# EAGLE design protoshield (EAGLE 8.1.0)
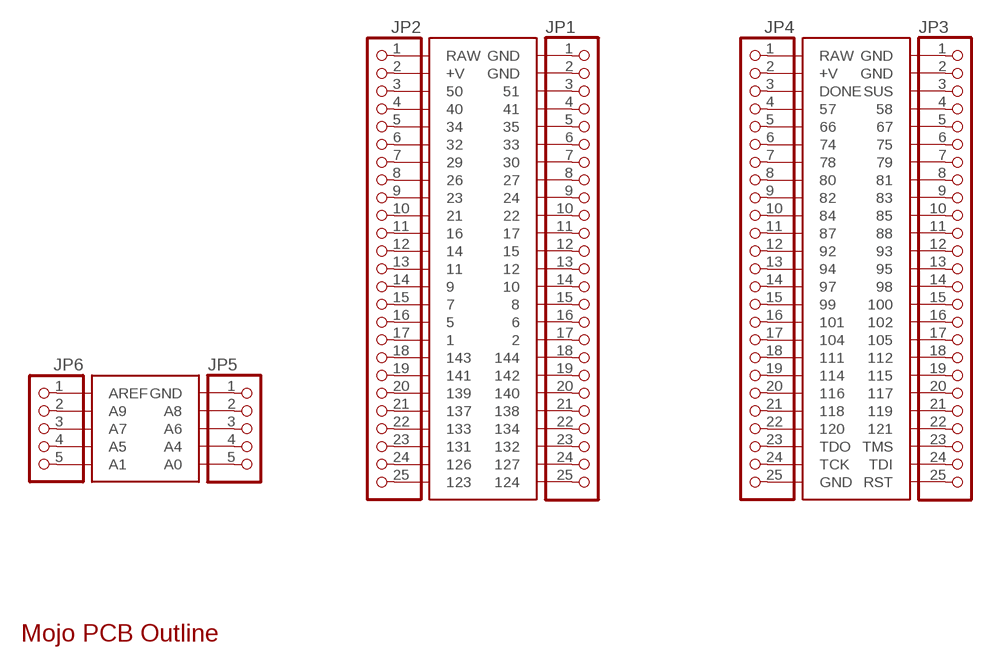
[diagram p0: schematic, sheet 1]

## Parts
JP1  PINHD-1X25  [1X25]
JP2  PINHD-1X25  [1X25]
JP3  PINHD-1X25  [1X25]
JP4  PINHD-1X25  [1X25]
JP5  PINHD-1X5MOJO  [1X5]
JP6  PINHD-1X5MOJO  [1X5]
U$1  MOJO_V2V3_NO_LABEL  [MOJO_V3_NO_LABEL]
U$2  MOJO_OUTLINE  [MOJO_OUTLINE]

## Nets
N$1: JP5.1 U$1.GND@5(GND)
N$2: JP5.2 U$1.A8
N$3: JP5.3 U$1.A6
N$4: JP5.4 U$1.A4
N$5: JP5.5 U$1.A0
N$6: JP6.1 U$1.AREF
N$7: JP6.2 U$1.A9
N$8: JP6.3 U$1.A7
N$9: JP6.4 U$1.A5
N$10: JP6.5 U$1.A1
N$11: JP1.1 U$1.GND@1(GND)
N$12: JP1.2 U$1.GND@2(GND)
N$13: JP1.3 U$1.51
N$14: JP1.4 U$1.41
N$15: JP1.5 U$1.35
N$16: JP1.6 U$1.33
N$17: JP1.7 U$1.30
N$18: JP1.8 U$1.27
N$19: JP1.9 U$1.24
N$20: JP1.10 U$1.22
N$21: JP1.11 U$1.17
N$22: JP1.12 U$1.15
N$23: JP1.13 U$1.12
N$24: JP1.14 U$1.10
N$25: JP1.15 U$1.8
N$26: JP1.16 U$1.6
N$27: JP1.17 U$1.2
N$28: JP1.18 U$1.144
N$29: JP1.19 U$1.142
N$30: JP1.20 U$1.140
N$31: JP1.21 U$1.138
N$32: JP1.22 U$1.134
N$33: JP1.23 U$1.132
N$34: JP1.24 U$1.127
N$35: JP1.25 U$1.124
N$36: JP2.1 U$1.RAW@1(RAW)
N$37: JP2.2 U$1.V@1(+V)
N$38: JP2.3 U$1.50
N$39: JP2.4 U$1.40
N$40: JP2.5 U$1.34
N$41: JP2.6 U$1.32
N$42: JP2.7 U$1.29
N$43: JP2.8 U$1.26
N$44: JP2.9 U$1.23
N$45: JP2.10 U$1.21
N$46: JP2.11 U$1.16
N$47: JP2.12 U$1.14
N$48: JP2.13 U$1.11
N$49: JP2.14 U$1.9
N$50: JP2.15 U$1.7
N$51: JP2.16 U$1.5
N$52: JP2.17 U$1.1
N$53: JP2.18 U$1.143
N$54: JP2.19 U$1.141
N$55: JP2.20 U$1.139
N$56: JP2.21 U$1.137
N$57: JP2.22 U$1.133
N$58: JP2.23 U$1.131
N$59: JP2.24 U$1.126
N$60: JP2.25 U$1.123
N$61: JP3.1 U$1.GND@3(GND)
N$62: JP3.2 U$1.GND@4(GND)
N$63: JP3.3 U$1.SUS
N$64: JP3.4 U$1.58
N$65: JP3.5 U$1.67
N$66: JP3.6 U$1.75
N$67: JP3.7 U$1.79
N$68: JP3.8 U$1.81
N$69: JP3.9 U$1.83
N$70: JP3.10 U$1.85
N$71: JP3.11 U$1.88
N$72: JP3.12 U$1.93
N$73: JP3.13 U$1.95
N$74: JP3.14 U$1.98
N$75: JP3.15 U$1.100
N$76: JP3.16 U$1.102
N$77: JP3.17 U$1.105
N$78: JP3.18 U$1.112
N$79: JP3.19 U$1.115
N$80: JP3.20 U$1.117
N$81: JP3.21 U$1.119
N$82: JP3.22 U$1.121
N$83: JP3.23 U$1.TMS
N$84: JP3.24 U$1.TDI
N$85: JP3.25 U$1.RST
N$86: JP4.1 U$1.RAW@2(RAW)
N$87: JP4.2 U$1.V@2(+V)
N$88: JP4.3 U$1.DONE
N$89: JP4.4 U$1.57
N$90: JP4.5 U$1.66
N$91: JP4.6 U$1.74
N$92: JP4.7 U$1.78
N$93: JP4.8 U$1.80
N$94: JP4.9 U$1.82
N$95: JP4.10 U$1.84
N$96: JP4.11 U$1.87
N$97: JP4.12 U$1.92
N$98: JP4.13 U$1.94
N$99: JP4.14 U$1.97
N$100: JP4.15 U$1.99
N$101: JP4.16 U$1.101
N$102: JP4.17 U$1.104
N$103: JP4.18 U$1.111
N$104: JP4.19 U$1.114
N$105: JP4.20 U$1.116
N$106: JP4.21 U$1.118
N$107: JP4.22 U$1.120
N$108: JP4.23 U$1.TDO
N$109: JP4.24 U$1.TCK
N$110: JP4.25 U$1.GND@6(GND)

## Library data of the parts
JP1-JP4 = embeddedmicro:PINHD-1X25: PIN HEADER
JP5 JP6 = embeddedmicro:PINHD-1X5: PIN HEADER
U$1 = embeddedmicro:MOJO_V2
U$2 = embeddedmicro:MOJO_OUTLINE

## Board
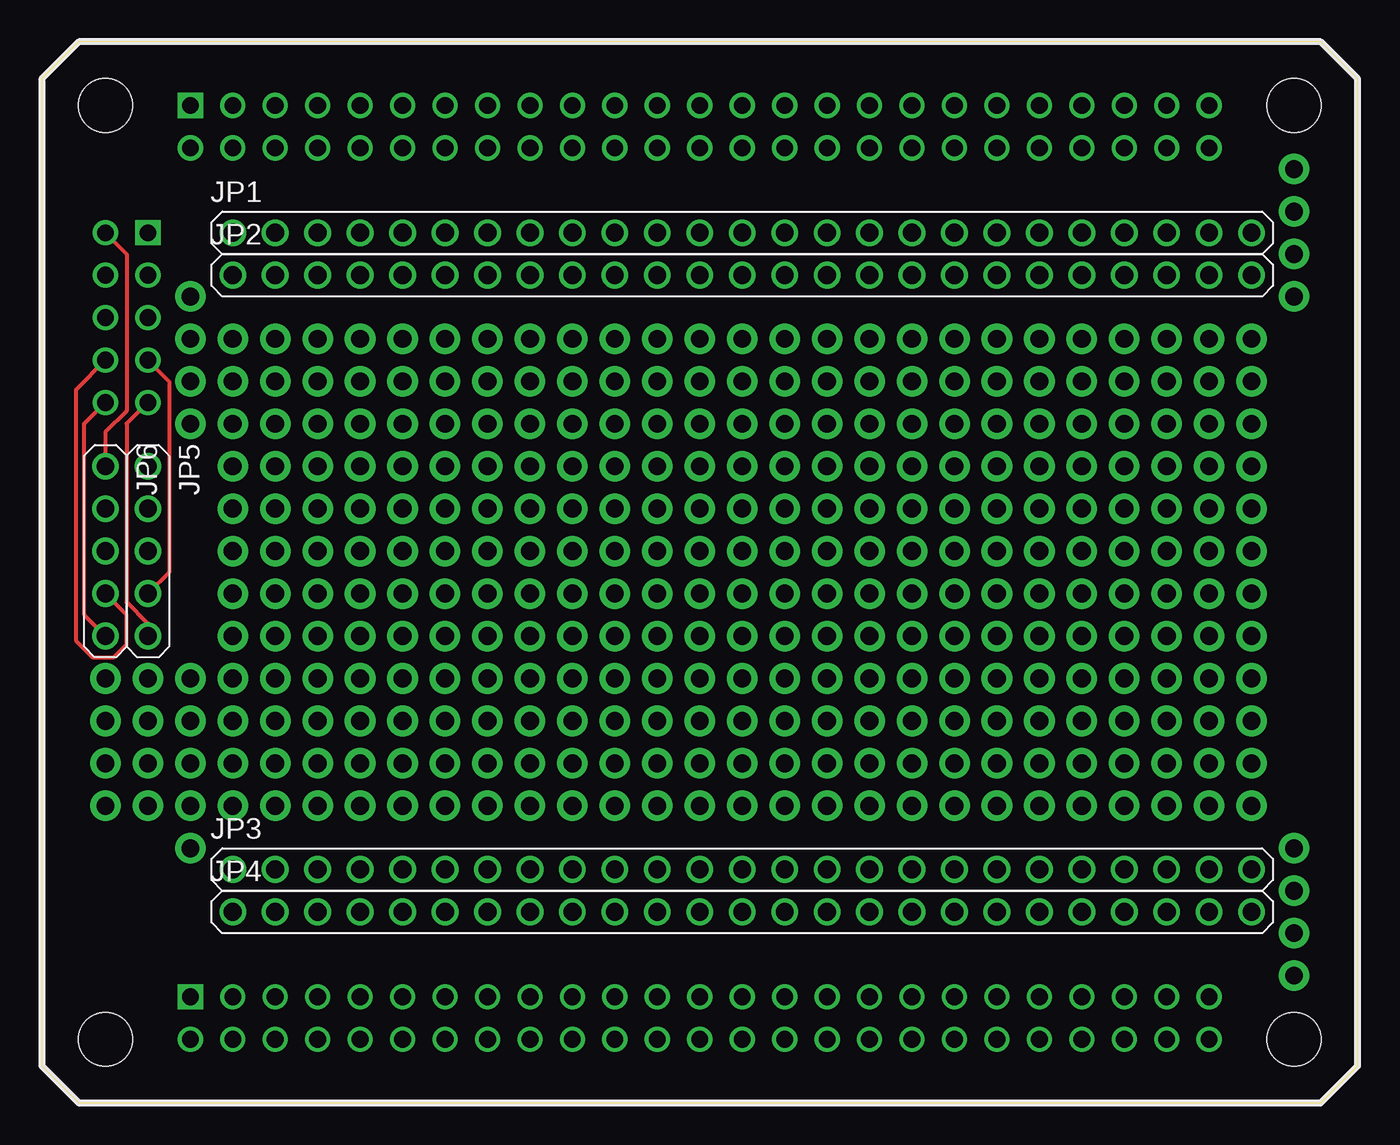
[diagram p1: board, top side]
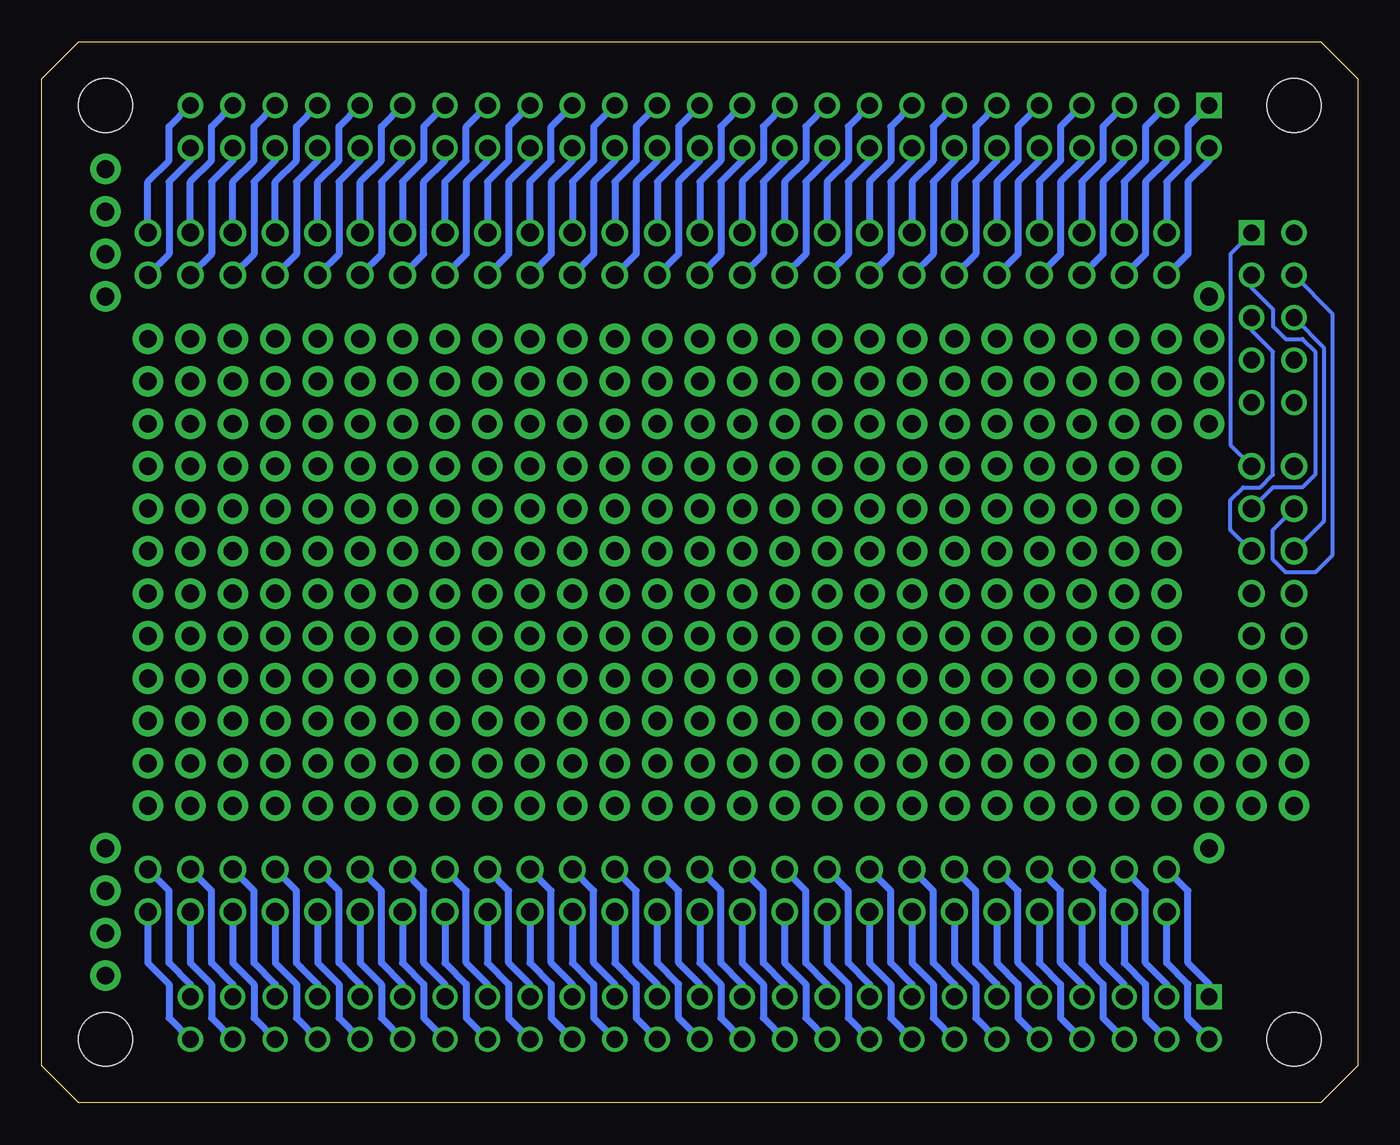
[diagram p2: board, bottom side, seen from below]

Size 78.74 x 63.5 mm. Coordinates in mm from the lower left corner, seen from the top.
Copper layers (1*16): Top 0.035mm / dielectric 1.5mm / Bottom 0.035mm
Design rules "default *": minimum track width 10mil, minimum drill 24mil, track to track 8mil, track to pad 8mil, pad to pad 8mil, via to via 8mil, smd to smd 8mil, copper to edge 40mil, drill to drill 8mil, minimum pad ring 10mil, minimum via ring 15mil, stop-mask expansion 4mil, vias tented up to drill 0mil, thermal gap 10mil

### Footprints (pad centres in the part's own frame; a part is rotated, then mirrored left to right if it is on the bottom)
1X25 = drill 1.067: 1 -29.21,0; 2 -26.67,0; 3 -24.13,0; 4 -21.59,0; 5 -19.05,0; 6 -16.51,0; 7 -13.97,0; 8 -11.43,0; 9 -8.89,0; 10 -6.35,0; 11 -3.81,0; 12 -1.27,0; 13 1.27,0; 14 3.81,0; 15 6.35,0; 16 8.89,0; 17 11.43,0; 18 13.97,0; 19 16.51,0; 20 19.05,0; 21 21.59,0; 22 24.13,0; 23 26.67,0; 24 29.21,0; 25 31.75,0
1X5 = drill 1.067: 1 -5.08,0; 2 -2.54,0; 3 0,0; 4 2.54,0; 5 5.08,0
MOJO_V3_NO_LABEL = drill 1: 1 49.53,57.15; 2 49.53,59.69; 5 46.99,57.15; 6 46.99,59.69; 7 44.45,57.15; 8 44.45,59.69; 9 41.91,57.15; 10 41.91,59.69; 11 39.37,57.15; 12 39.37,59.69; 14 36.83,57.15; 15 36.83,59.69; 16 34.29,57.15; 17 34.29,59.69; 21 31.75,57.15; 22 31.75,59.69; 23 29.21,57.15; 24 29.21,59.69; 26 26.67,57.15; 27 26.67,59.69; 29 24.13,57.15; 30 24.13,59.69; 32 21.59,57.15; 33 21.59,59.69; 34 19.05,57.15; 35 19.05,59.69; 40 16.51,57.15; 41 16.51,59.69; 50 13.97,57.15; 51 13.97,59.69; 57 16.51,3.81; 58 16.51,6.35; 66 19.05,3.81; 67 19.05,6.35; 74 21.59,3.81; 75 21.59,6.35; 78 24.13,3.81; 79 24.13,6.35; 80 26.67,3.81; 81 26.67,6.35; 82 29.21,3.81; 83 29.21,6.35; 84 31.75,3.81; 85 31.75,6.35; 87 34.29,3.81; 88 34.29,6.35; 92 36.83,3.81; 93 36.83,6.35; 94 39.37,3.81; 95 39.37,6.35; 97 41.91,3.81; 98 41.91,6.35; 99 44.45,3.81; 100 44.45,6.35; 101 46.99,3.81; 102 46.99,6.35; 104 49.53,3.81; 105 49.53,6.35; 111 52.07,3.81; 112 52.07,6.35; 114 54.61,3.81; 115 54.61,6.35; 116 57.15,3.81; 117 57.15,6.35; 118 59.69,3.81; 119 59.69,6.35; 120 62.23,3.81; 121 62.23,6.35; 123 69.85,57.15; 124 69.85,59.69; 126 67.31,57.15; 127 67.31,59.69; 131 64.77,57.15; 132 64.77,59.69; 133 62.23,57.15; 134 62.23,59.69; 137 59.69,57.15; 138 59.69,59.69; 139 57.15,57.15; 140 57.15,59.69; 141 54.61,57.15; 142 54.61,59.69; 143 52.07,57.15; 144 52.07,59.69; A0 6.35,41.91; A1 3.81,41.91; A4 6.35,44.45; A5 3.81,44.45; A6 6.35,46.99; A7 3.81,46.99; A8 6.35,49.53; A9 3.81,49.53; AREF 3.81,52.07; DONE 13.97,3.81; GND@2 11.43,59.69; GND@4 11.43,6.35; GND@6 69.85,3.81; RAW@1 8.89,57.15; RAW@2 8.89,3.81; RST 69.85,6.35; SUS 13.97,6.35; TCK 67.31,3.81; TDI 67.31,6.35; TDO 64.77,3.81; TMS 64.77,6.35; V@1 11.43,57.15; V@2 11.43,3.81 | drill 1 square: GND@1 8.89,59.69; GND@3 8.89,6.35; GND@5 6.35,52.07 | hole 3.2: 3.81,3.81; 3.81,59.69; 74.93,59.69; 74.93,3.81

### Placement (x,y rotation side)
JP1  40.64,52.07 0 top
JP2  40.64,49.53 0 top
JP3  40.64,13.97 0 top
JP4  40.64,11.43 0 top
JP5  6.35,33.02 270 top
JP6  3.81,33.02 270 top
U$1  0,0 0 top
U$2  0,0 0 top

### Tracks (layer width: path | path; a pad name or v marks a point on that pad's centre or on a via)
N$1
  Bottom 0.254: U$1.GND@5 7.62,50.8 7.62,39.37 JP5.1
N$2
  Bottom 0.254: U$1.A8 6.35,48.77 5.08,47.5 5.08,46.48 4.32,45.72 3.3,45.72 2.54,44.96 2.54,37.59 3.3,36.83 5.08,36.83 JP5.2
N$3
  Bottom 0.254: JP5.3 7.62,34.29 7.62,36.07 6.86,36.83 5.84,36.83 5.08,37.59 5.08,44.96 6.35,46.23 U$1.A6
N$4
  Top 0.254: U$1.A4 7.62,43.18 7.62,31.75 JP5.4
N$5
  Top 0.254: U$1.A0 5.08,40.64 5.08,29.97 6.35,28.7 JP5.5
N$6
  Top 0.254: U$1.AREF 4.83,51.05 5.08,50.8 5.08,41.4 3.81,40.13 JP6.1
N$7
  Bottom 0.254: U$1.A9 1.52,47.24 1.52,32.77 2.54,31.75 4.32,31.75 5.08,32.51 5.08,34.29 JP6.2
N$8
  Bottom 0.254: U$1.A7 2.03,45.21 2.03,34.8 JP6.3
N$9
  Top 0.254: U$1.A5 2.03,42.67 2.03,27.69 3.05,26.67 4.32,26.67 5.08,27.43 5.08,29.21 JP6.4
N$10
  Top 0.254: U$1.A1 2.54,40.64 2.54,29.21 JP6.5
N$11
  Bottom 0.406: U$1.GND@1 10.16,58.42 10.16,56.39 11.43,55.12 JP1.1
N$12
  Bottom 0.406: U$1.GND@2 12.7,58.42 12.7,56.39 13.97,55.12 JP1.2
N$13
  Bottom 0.406: U$1.51 15.24,58.42 15.24,56.39 16.51,55.12 JP1.3
N$14
  Bottom 0.406: U$1.41 17.78,58.42 17.78,56.39 19.05,55.12 JP1.4
N$15
  Bottom 0.406: U$1.35 20.32,58.42 20.32,56.39 21.59,55.12 JP1.5
N$16
  Bottom 0.406: U$1.33 22.86,58.42 22.86,56.39 24.13,55.12 JP1.6
N$17
  Bottom 0.406: U$1.30 25.4,58.42 25.4,56.39 26.67,55.12 JP1.7
N$18
  Bottom 0.406: U$1.27 27.94,58.42 27.94,56.39 29.21,55.12 JP1.8
N$19
  Bottom 0.406: U$1.24 30.48,58.42 30.48,56.39 31.75,55.12 JP1.9
N$20
  Bottom 0.406: U$1.22 33.02,58.42 33.02,56.39 34.29,55.12 JP1.10
N$21
  Bottom 0.406: U$1.17 35.56,58.42 35.56,56.39 36.83,55.12 JP1.11
N$22
  Bottom 0.406: U$1.15 38.1,58.42 38.1,56.39 39.37,55.12 JP1.12
N$23
  Bottom 0.406: U$1.12 40.64,58.42 40.64,56.39 41.91,55.12 JP1.13
N$24
  Bottom 0.406: U$1.10 43.18,58.42 43.18,56.39 44.45,55.12 JP1.14
N$25
  Bottom 0.406: U$1.8 45.72,58.42 45.72,56.39 46.99,55.12 JP1.15
N$26
  Bottom 0.406: JP1.16 49.53,55.12 48.26,56.39 48.26,58.42 U$1.6
N$27
  Bottom 0.406: U$1.2 50.8,58.42 50.8,56.39 52.07,55.12 JP1.17
N$28
  Bottom 0.406: JP1.18 54.61,55.12 53.34,56.39 53.34,58.42 U$1.144
N$29
  Bottom 0.406: U$1.142 55.88,58.42 55.88,56.39 57.15,55.12 JP1.19
N$30
  Bottom 0.406: JP1.20 59.69,55.12 58.42,56.39 58.42,58.42 U$1.140
N$31
  Bottom 0.406: JP1.21 62.23,55.12 60.96,56.39 60.96,58.42 U$1.138
N$32
  Bottom 0.406: JP1.22 64.77,55.12 63.5,56.39 63.5,58.42 U$1.134
N$33
  Bottom 0.406: JP1.23 67.31,55.12 66.04,56.39 66.04,58.42 U$1.132
N$34
  Bottom 0.406: JP1.24 69.85,55.12 68.58,56.39 68.58,58.42 U$1.127
N$35
  Bottom 0.406: JP1.25 72.39,55.12 71.12,56.39 71.12,58.42 U$1.124
N$36
  Bottom 0.406: U$1.RAW@1 8.89,56.39 10.16,55.12 10.16,50.8 JP2.1
N$37
  Bottom 0.406: U$1.V@1 11.43,56.39 12.7,55.12 12.7,50.8 JP2.2
N$38
  Bottom 0.406: U$1.50 13.97,56.39 15.24,55.12 15.24,50.8 JP2.3
N$39
  Bottom 0.406: U$1.40 16.51,56.39 17.78,55.12 17.78,50.8 JP2.4
N$40
  Bottom 0.406: U$1.34 19.05,56.39 20.32,55.12 20.32,50.8 JP2.5
N$41
  Bottom 0.406: U$1.32 21.59,56.39 22.86,55.12 22.86,50.8 JP2.6
N$42
  Bottom 0.406: U$1.29 24.13,56.39 25.4,55.12 25.4,50.8 JP2.7
N$43
  Bottom 0.406: U$1.26 26.67,56.39 27.94,55.12 27.94,50.8 JP2.8
N$44
  Bottom 0.406: U$1.23 29.21,56.39 30.23,55.37 30.48,55.12 30.48,50.8 JP2.9
N$45
  Bottom 0.406: U$1.21 31.75,56.39 33.02,55.12 33.02,50.8 JP2.10
N$46
  Bottom 0.406: U$1.16 34.29,56.39 35.31,55.37 35.56,55.12 35.56,50.8 JP2.11
N$47
  Bottom 0.406: U$1.14 36.83,56.39 38.1,55.12 38.1,50.8 JP2.12
N$48
  Bottom 0.406: U$1.11 39.37,56.39 40.64,55.12 40.64,50.8 JP2.13
N$49
  Bottom 0.406: U$1.9 41.91,56.39 43.18,55.12 43.18,50.8 JP2.14
N$50
  Bottom 0.406: U$1.7 44.45,56.39 45.72,55.12 45.72,50.8 JP2.15
N$51
  Bottom 0.406: U$1.5 46.99,56.39 48.26,55.12 48.26,50.8 JP2.16
N$52
  Bottom 0.406: U$1.1 49.53,56.39 50.8,55.12 50.8,50.8 JP2.17
N$53
  Bottom 0.406: U$1.143 52.07,56.39 53.34,55.12 53.34,50.8 JP2.18
N$54
  Bottom 0.406: JP2.19 55.88,50.8 55.88,55.12 54.61,56.39 U$1.141
N$55
  Bottom 0.406: U$1.139 57.15,56.39 58.17,55.37 58.42,55.12 58.42,50.8 JP2.20
N$56
  Bottom 0.406: U$1.137 59.69,56.39 60.96,55.12 60.96,50.8 JP2.21
N$57
  Bottom 0.406: U$1.133 62.23,56.39 63.5,55.12 63.5,50.8 JP2.22
N$58
  Bottom 0.406: U$1.131 64.77,56.39 66.04,55.12 66.04,50.8 JP2.23
N$59
  Bottom 0.406: U$1.126 67.31,56.39 68.58,55.12 68.58,50.8 JP2.24
N$60
  Bottom 0.406: U$1.123 69.85,56.39 71.12,55.12 71.12,50.8 JP2.25
N$61
  Bottom 0.406: U$1.GND@3 8.89,7.11 10.16,8.38 10.16,12.7 JP3.1
N$62
  Bottom 0.406: U$1.GND@4 11.43,7.11 12.7,8.38 12.7,12.7 JP3.2
N$63
  Bottom 0.406: U$1.SUS 13.97,7.11 15.24,8.38 15.24,12.7 JP3.3
N$64
  Bottom 0.406: U$1.58 16.51,7.11 17.78,8.38 17.78,12.7 JP3.4
N$65
  Bottom 0.406: U$1.67 19.05,7.11 20.32,8.38 20.32,12.7 JP3.5
N$66
  Bottom 0.406: U$1.75 21.59,7.11 22.86,8.38 22.86,12.7 JP3.6
N$67
  Bottom 0.406: U$1.79 24.13,7.11 25.4,8.38 25.4,12.7 JP3.7
N$68
  Bottom 0.406: U$1.81 26.67,7.11 27.94,8.38 27.94,12.7 JP3.8
N$69
  Bottom 0.406: U$1.83 29.21,7.11 30.48,8.38 30.48,12.7 JP3.9
N$70
  Bottom 0.406: U$1.85 31.75,7.11 33.02,8.38 33.02,12.7 JP3.10
N$71
  Bottom 0.406: U$1.88 34.29,7.11 35.56,8.38 35.56,12.7 JP3.11
N$72
  Bottom 0.406: U$1.93 36.83,7.11 38.1,8.38 38.1,12.7 JP3.12
N$73
  Bottom 0.406: U$1.95 39.37,7.11 40.39,8.13 40.64,8.38 40.64,12.7 JP3.13
N$74
  Bottom 0.406: U$1.98 41.91,7.11 43.18,8.38 43.18,12.7 JP3.14
N$75
  Bottom 0.406: U$1.100 44.45,7.11 45.72,8.38 45.72,12.7 JP3.15
N$76
  Bottom 0.406: U$1.102 46.99,7.11 48.26,8.38 48.26,12.7 JP3.16
N$77
  Bottom 0.406: U$1.105 49.53,7.11 50.8,8.38 50.8,12.7 JP3.17
N$78
  Bottom 0.406: U$1.112 52.07,7.11 53.34,8.38 53.34,12.7 JP3.18
N$79
  Bottom 0.406: U$1.115 54.61,7.11 55.88,8.38 55.88,12.7 JP3.19
N$80
  Bottom 0.406: U$1.117 57.15,7.11 58.42,8.38 58.42,12.7 JP3.20
N$81
  Bottom 0.406: U$1.119 59.69,7.11 60.96,8.38 60.96,12.7 JP3.21
N$82
  Bottom 0.406: U$1.121 62.23,7.11 63.25,8.13 63.5,8.38 63.5,12.7 JP3.22
N$83
  Bottom 0.406: U$1.TMS 64.77,7.11 66.04,8.38 66.04,12.7 JP3.23
N$84
  Bottom 0.406: U$1.TDI 67.31,7.11 68.58,8.38 68.58,12.7 JP3.24
N$85
  Bottom 0.406: U$1.RST 69.85,7.11 71.12,8.38 71.12,12.7 JP3.25
N$86
  Bottom 0.406: U$1.RAW@2 10.16,5.08 10.16,7.11 11.43,8.38 JP4.1
N$87
  Bottom 0.406: JP4.2 13.97,8.38 12.7,7.11 12.7,5.08 U$1.V@2
N$88
  Bottom 0.406: JP4.3 16.51,8.38 15.24,7.11 15.24,5.08 U$1.DONE
N$89
  Bottom 0.406: JP4.4 19.05,8.38 17.78,7.11 17.78,5.08 U$1.57
N$90
  Bottom 0.406: JP4.5 21.59,8.38 20.32,7.11 20.32,5.08 U$1.66
N$91
  Bottom 0.406: JP4.6 24.13,8.38 22.86,7.11 22.86,5.08 U$1.74
N$92
  Bottom 0.406: JP4.7 26.67,8.38 25.4,7.11 25.4,5.08 U$1.78
N$93
  Bottom 0.406: JP4.8 29.21,8.38 27.94,7.11 27.94,5.08 U$1.80
N$94
  Bottom 0.406: JP4.9 31.75,8.38 30.48,7.11 30.48,5.08 U$1.82
N$95
  Bottom 0.406: JP4.10 34.29,8.38 33.02,7.11 33.02,5.08 U$1.84
N$96
  Bottom 0.406: JP4.11 36.83,8.38 35.56,7.11 35.56,5.08 U$1.87
N$97
  Bottom 0.406: JP4.12 39.37,8.38 38.1,7.11 38.1,5.08 U$1.92
N$98
  Bottom 0.406: U$1.94 40.64,5.08 40.64,7.11 41.91,8.38 JP4.13
N$99
  Bottom 0.406: JP4.14 44.45,8.38 43.18,7.11 43.18,5.08 U$1.97
N$100
  Bottom 0.406: JP4.15 46.99,8.38 45.72,7.11 45.72,5.08 U$1.99
N$101
  Bottom 0.406: JP4.16 49.53,8.38 48.26,7.11 48.26,5.08 U$1.101
N$102
  Bottom 0.406: JP4.17 52.07,8.38 50.8,7.11 50.8,5.08 U$1.104
N$103
  Bottom 0.406: JP4.18 54.61,8.38 53.34,7.11 53.34,5.08 U$1.111
N$104
  Bottom 0.406: JP4.19 57.15,8.38 55.88,7.11 55.88,5.08 U$1.114
N$105
  Bottom 0.406: JP4.20 59.69,8.38 58.42,7.11 58.42,5.08 U$1.116
N$106
  Bottom 0.406: JP4.21 62.23,8.38 60.96,7.11 60.96,5.08 U$1.118
N$107
  Bottom 0.406: JP4.22 64.77,8.38 63.5,7.11 63.5,5.08 U$1.120
N$108
  Bottom 0.406: JP4.23 67.31,8.38 66.04,7.11 66.04,5.08 U$1.TDO
N$109
  Bottom 0.406: JP4.24 69.85,8.38 68.58,7.11 68.58,5.08 U$1.TCK
N$110
  Bottom 0.406: JP4.25 72.39,8.38 71.12,7.11 71.12,5.08 U$1.GND@6
N$111  (via drill 1.07)
  other vias: 21.59,45.72
N$112  (via drill 1.07)
  other vias: 11.43,43.18
N$113  (via drill 1.07)
  other vias: 11.43,45.72
N$114  (via drill 1.07)
  other vias: 13.97,45.72
N$115  (via drill 1.07)
  other vias: 16.51,45.72
N$116  (via drill 1.07)
  other vias: 19.05,45.72
N$117  (via drill 1.07)
  other vias: 24.13,45.72
N$118  (via drill 1.07)
  other vias: 26.67,45.72
N$119  (via drill 1.07)
  other vias: 29.21,45.72
N$120  (via drill 1.07)
  other vias: 31.75,45.72
N$121  (via drill 1.07)
  other vias: 34.29,45.72
N$122  (via drill 1.07)
  other vias: 36.83,45.72
N$123  (via drill 1.07)
  other vias: 39.37,45.72
N$124  (via drill 1.07)
  other vias: 41.91,45.72
N$125  (via drill 1.07)
  other vias: 44.45,45.72
N$126  (via drill 1.07)
  other vias: 46.99,45.72
N$127  (via drill 1.07)
  other vias: 49.53,45.72
N$128  (via drill 1.07)
  other vias: 52.07,45.72
N$129  (via drill 1.07)
  other vias: 54.61,45.72
N$130  (via drill 1.07)
  other vias: 57.15,45.72
N$131  (via drill 1.07)
  other vias: 59.69,45.72
N$132  (via drill 1.07)
  other vias: 62.23,45.72
N$133  (via drill 1.07)
  other vias: 64.77,45.72
N$134  (via drill 1.07)
  other vias: 67.31,45.72
N$135  (via drill 1.07)
  other vias: 69.85,45.72
N$136  (via drill 1.07)
  other vias: 72.39,45.72
N$137  (via drill 1.07)
  other vias: 13.97,43.18
N$138  (via drill 1.07)
  other vias: 16.51,43.18
N$139  (via drill 1.07)
  other vias: 19.05,43.18
N$140  (via drill 1.07)
  other vias: 21.59,43.18
N$141  (via drill 1.07)
  other vias: 24.13,43.18
N$142  (via drill 1.07)
  other vias: 26.67,43.18
N$143  (via drill 1.07)
  other vias: 29.21,43.18
N$144  (via drill 1.07)
  other vias: 31.75,43.18
N$145  (via drill 1.07)
  other vias: 34.29,43.18
N$146  (via drill 1.07)
  other vias: 36.83,43.18
N$147  (via drill 1.07)
  other vias: 39.37,43.18
N$148  (via drill 1.07)
  other vias: 41.91,43.18
N$149  (via drill 1.07)
  other vias: 44.45,43.18
N$150  (via drill 1.07)
  other vias: 46.99,43.18
N$151  (via drill 1.07)
  other vias: 49.53,43.18
N$152  (via drill 1.07)
  other vias: 52.07,43.18
N$153  (via drill 1.07)
  other vias: 54.61,43.18
N$154  (via drill 1.07)
  other vias: 57.15,43.18
N$155  (via drill 1.07)
  other vias: 59.69,43.18
N$156  (via drill 1.07)
  other vias: 62.23,43.18
N$157  (via drill 1.07)
  other vias: 64.77,43.18
N$158  (via drill 1.07)
  other vias: 67.31,43.18
N$159  (via drill 1.07)
  other vias: 69.85,43.18
N$160  (via drill 1.07)
  other vias: 72.39,43.18
N$161  (via drill 1.07)
  other vias: 11.43,40.64
N$162  (via drill 1.07)
  other vias: 13.97,40.64
N$163  (via drill 1.07)
  other vias: 16.51,40.64
N$164  (via drill 1.07)
  other vias: 19.05,40.64
N$165  (via drill 1.07)
  other vias: 21.59,40.64
N$166  (via drill 1.07)
  other vias: 24.13,40.64
N$167  (via drill 1.07)
  other vias: 26.67,40.64
N$168  (via drill 1.07)
  other vias: 29.21,40.64
N$169  (via drill 1.07)
  other vias: 31.75,40.64
N$170  (via drill 1.07)
  other vias: 34.29,40.64
N$171  (via drill 1.07)
  other vias: 36.83,40.64
N$172  (via drill 1.07)
  other vias: 39.37,40.64
N$173  (via drill 1.07)
  other vias: 41.91,40.64
N$174  (via drill 1.07)
  other vias: 44.45,40.64
N$175  (via drill 1.07)
  other vias: 46.99,40.64
N$176  (via drill 1.07)
  other vias: 49.53,40.64
N$177  (via drill 1.07)
  other vias: 52.07,40.64
N$178  (via drill 1.07)
  other vias: 54.61,40.64
N$179  (via drill 1.07)
  other vias: 57.15,40.64
N$180  (via drill 1.07)
  other vias: 59.69,40.64
N$181  (via drill 1.07)
  other vias: 62.23,40.64
N$182  (via drill 1.07)
  other vias: 64.77,40.64
N$183  (via drill 1.07)
  other vias: 67.31,40.64
N$184  (via drill 1.07)
  other vias: 69.85,40.64
N$185  (via drill 1.07)
  other vias: 72.39,40.64
N$186  (via drill 1.07)
  other vias: 11.43,38.1
N$187  (via drill 1.07)
  other vias: 13.97,38.1
N$188  (via drill 1.07)
  other vias: 16.51,38.1
N$189  (via drill 1.07)
  other vias: 19.05,38.1
N$190  (via drill 1.07)
  other vias: 21.59,38.1
N$191  (via drill 1.07)
  other vias: 24.13,38.1
N$192  (via drill 1.07)
  other vias: 26.67,38.1
N$193  (via drill 1.07)
  other vias: 29.21,38.1
N$194  (via drill 1.07)
  other vias: 31.75,38.1
N$195  (via drill 1.07)
  other vias: 34.29,38.1
N$196  (via drill 1.07)
  other vias: 36.83,38.1
N$197  (via drill 1.07)
  other vias: 39.37,38.1
N$198  (via drill 1.07)
  other vias: 41.91,38.1
N$199  (via drill 1.07)
  other vias: 44.45,38.1
N$200  (via drill 1.07)
  other vias: 46.99,38.1
N$201  (via drill 1.07)
  other vias: 49.53,38.1
N$202  (via drill 1.07)
  other vias: 52.07,38.1
N$203  (via drill 1.07)
  other vias: 54.61,38.1
N$204  (via drill 1.07)
  other vias: 57.15,38.1
N$205  (via drill 1.07)
  other vias: 59.69,38.1
N$206  (via drill 1.07)
  other vias: 62.23,38.1
N$207  (via drill 1.07)
  other vias: 64.77,38.1
N$208  (via drill 1.07)
  other vias: 67.31,38.1
N$209  (via drill 1.07)
  other vias: 69.85,38.1
N$210  (via drill 1.07)
  other vias: 72.39,38.1
N$211  (via drill 1.07)
  other vias: 8.89,15.24
N$212  (via drill 1.07)
  other vias: 13.97,35.56
N$213  (via drill 1.07)
  other vias: 16.51,35.56
N$214  (via drill 1.07)
  other vias: 19.05,35.56
N$215  (via drill 1.07)
  other vias: 21.59,35.56
N$216  (via drill 1.07)
  other vias: 24.13,35.56
N$217  (via drill 1.07)
  other vias: 26.67,35.56
N$218  (via drill 1.07)
  other vias: 29.21,35.56
N$219  (via drill 1.07)
  other vias: 31.75,35.56
N$220  (via drill 1.07)
  other vias: 34.29,35.56
N$221  (via drill 1.07)
  other vias: 36.83,35.56
N$222  (via drill 1.07)
  other vias: 39.37,35.56
N$223  (via drill 1.07)
  other vias: 41.91,35.56
N$224  (via drill 1.07)
  other vias: 44.45,35.56
N$225  (via drill 1.07)
  other vias: 46.99,35.56
N$226  (via drill 1.07)
  other vias: 49.53,35.56
N$227  (via drill 1.07)
  other vias: 52.07,35.56
N$228  (via drill 1.07)
  other vias: 54.61,35.56
N$229  (via drill 1.07)
  other vias: 57.15,35.56
N$230  (via drill 1.07)
  other vias: 59.69,35.56
N$231  (via drill 1.07)
  other vias: 62.23,35.56
N$232  (via drill 1.07)
  other vias: 64.77,35.56
N$233  (via drill 1.07)
  other vias: 67.31,35.56
N$234  (via drill 1.07)
  other vias: 69.85,35.56
N$235  (via drill 1.07)
  other vias: 72.39,35.56
N$236  (via drill 1.07)
  other vias: 11.43,33.02
N$237  (via drill 1.07)
  other vias: 13.97,33.02
N$238  (via drill 1.07)
  other vias: 16.51,33.02
N$239  (via drill 1.07)
  other vias: 19.05,33.02
N$240  (via drill 1.07)
  other vias: 21.59,33.02
N$241  (via drill 1.07)
  other vias: 24.13,33.02
N$242  (via drill 1.07)
  other vias: 26.67,33.02
N$243  (via drill 1.07)
  other vias: 29.21,33.02
N$244  (via drill 1.07)
  other vias: 31.75,33.02
N$245  (via drill 1.07)
  other vias: 34.29,33.02
N$246  (via drill 1.07)
  other vias: 36.83,33.02
N$247  (via drill 1.07)
  other vias: 39.37,33.02
N$248  (via drill 1.07)
  other vias: 41.91,33.02
N$249  (via drill 1.07)
  other vias: 44.45,33.02
N$250  (via drill 1.07)
  other vias: 46.99,33.02
N$251  (via drill 1.07)
  other vias: 49.53,33.02
N$252  (via drill 1.07)
  other vias: 52.07,33.02
N$253  (via drill 1.07)
  other vias: 54.61,33.02
N$254  (via drill 1.07)
  other vias: 57.15,33.02
N$255  (via drill 1.07)
  other vias: 59.69,33.02
N$256  (via drill 1.07)
  other vias: 62.23,33.02
N$257  (via drill 1.07)
  other vias: 64.77,33.02
N$258  (via drill 1.07)
  other vias: 67.31,33.02
N$259  (via drill 1.07)
  other vias: 69.85,33.02
N$260  (via drill 1.07)
  other vias: 72.39,33.02
N$261  (via drill 1.07)
  other vias: 11.43,30.48
N$262  (via drill 1.07)
  other vias: 13.97,30.48
N$263  (via drill 1.07)
  other vias: 16.51,30.48
N$264  (via drill 1.07)
  other vias: 19.05,30.48
N$265  (via drill 1.07)
  other vias: 21.59,30.48
N$266  (via drill 1.07)
  other vias: 24.13,30.48
N$267  (via drill 1.07)
  other vias: 26.67,30.48
N$268  (via drill 1.07)
  other vias: 29.21,30.48
N$269  (via drill 1.07)
  other vias: 31.75,30.48
N$270  (via drill 1.07)
  other vias: 34.29,30.48
N$271  (via drill 1.07)
  other vias: 36.83,30.48
N$272  (via drill 1.07)
  other vias: 39.37,30.48
N$273  (via drill 1.07)
  other vias: 41.91,30.48
N$274  (via drill 1.07)
  other vias: 44.45,30.48
N$275  (via drill 1.07)
  other vias: 46.99,30.48
N$276  (via drill 1.07)
  other vias: 49.53,30.48
N$277  (via drill 1.07)
  other vias: 52.07,30.48
N$278  (via drill 1.07)
  other vias: 54.61,30.48
N$279  (via drill 1.07)
  other vias: 57.15,30.48
N$280  (via drill 1.07)
  other vias: 59.69,30.48
N$281  (via drill 1.07)
  other vias: 62.23,30.48
N$282  (via drill 1.07)
  other vias: 64.77,30.48
N$283  (via drill 1.07)
  other vias: 67.31,30.48
N$284  (via drill 1.07)
  other vias: 69.85,30.48
N$285  (via drill 1.07)
  other vias: 72.39,30.48
N$286  (via drill 1.07)
  other vias: 11.43,27.94
N$287  (via drill 1.07)
  other vias: 13.97,27.94
N$288  (via drill 1.07)
  other vias: 16.51,27.94
N$289  (via drill 1.07)
  other vias: 19.05,27.94
N$290  (via drill 1.07)
  other vias: 21.59,27.94
N$291  (via drill 1.07)
  other vias: 24.13,27.94
N$292  (via drill 1.07)
  other vias: 26.67,27.94
N$293  (via drill 1.07)
  other vias: 29.21,27.94
N$294  (via drill 1.07)
  other vias: 31.75,27.94
N$295  (via drill 1.07)
  other vias: 34.29,27.94
N$296  (via drill 1.07)
  other vias: 36.83,27.94
N$297  (via drill 1.07)
  other vias: 39.37,27.94
N$298  (via drill 1.07)
  other vias: 41.91,27.94
N$299  (via drill 1.07)
  other vias: 44.45,27.94
N$300  (via drill 1.07)
  other vias: 46.99,27.94
N$301  (via drill 1.07)
  other vias: 49.53,27.94
N$302  (via drill 1.07)
  other vias: 52.07,27.94
N$303  (via drill 1.07)
  other vias: 54.61,27.94
N$304  (via drill 1.07)
  other vias: 57.15,27.94
N$305  (via drill 1.07)
  other vias: 59.69,27.94
N$306  (via drill 1.07)
  other vias: 62.23,27.94
N$307  (via drill 1.07)
  other vias: 64.77,27.94
N$308  (via drill 1.07)
  other vias: 67.31,27.94
N$309  (via drill 1.07)
  other vias: 69.85,27.94
N$310  (via drill 1.07)
  other vias: 72.39,27.94
N$311  (via drill 1.07)
  other vias: 11.43,25.4
N$312  (via drill 1.07)
  other vias: 13.97,25.4
N$313  (via drill 1.07)
  other vias: 16.51,25.4
N$314  (via drill 1.07)
  other vias: 19.05,25.4
N$315  (via drill 1.07)
  other vias: 21.59,25.4
N$316  (via drill 1.07)
  other vias: 24.13,25.4
N$317  (via drill 1.07)
  other vias: 26.67,25.4
N$318  (via drill 1.07)
  other vias: 29.21,25.4
N$319  (via drill 1.07)
  other vias: 31.75,25.4
N$320  (via drill 1.07)
  other vias: 34.29,25.4
N$321  (via drill 1.07)
  other vias: 36.83,25.4
N$322  (via drill 1.07)
  other vias: 39.37,25.4
N$323  (via drill 1.07)
  other vias: 41.91,25.4
N$324  (via drill 1.07)
  other vias: 44.45,25.4
N$325  (via drill 1.07)
  other vias: 46.99,25.4
N$326  (via drill 1.07)
  other vias: 49.53,25.4
N$327  (via drill 1.07)
  other vias: 52.07,25.4
N$328  (via drill 1.07)
  other vias: 54.61,25.4
N$329  (via drill 1.07)
  other vias: 57.15,25.4
N$330  (via drill 1.07)
  other vias: 59.69,25.4
N$331  (via drill 1.07)
  other vias: 62.23,25.4
N$332  (via drill 1.07)
  other vias: 64.77,25.4
N$333  (via drill 1.07)
  other vias: 67.31,25.4
N$334  (via drill 1.07)
  other vias: 69.85,25.4
N$335  (via drill 1.07)
  other vias: 72.39,25.4
N$336  (via drill 1.07)
  other vias: 11.43,22.86
N$337  (via drill 1.07)
  other vias: 13.97,22.86
N$338  (via drill 1.07)
  other vias: 16.51,22.86
N$339  (via drill 1.07)
  other vias: 19.05,22.86
N$340  (via drill 1.07)
  other vias: 21.59,22.86
N$341  (via drill 1.07)
  other vias: 24.13,22.86
N$342  (via drill 1.07)
  other vias: 26.67,22.86
N$343  (via drill 1.07)
  other vias: 29.21,22.86
N$344  (via drill 1.07)
  other vias: 31.75,22.86
N$345  (via drill 1.07)
  other vias: 34.29,22.86
N$346  (via drill 1.07)
  other vias: 36.83,22.86
N$347  (via drill 1.07)
  other vias: 39.37,22.86
N$348  (via drill 1.07)
  other vias: 41.91,22.86
N$349  (via drill 1.07)
  other vias: 44.45,22.86
N$350  (via drill 1.07)
  other vias: 46.99,22.86
N$351  (via drill 1.07)
  other vias: 49.53,22.86
N$352  (via drill 1.07)
  other vias: 52.07,22.86
N$353  (via drill 1.07)
  other vias: 54.61,22.86
N$354  (via drill 1.07)
  other vias: 57.15,22.86
N$355  (via drill 1.07)
  other vias: 59.69,22.86
N$356  (via drill 1.07)
  other vias: 62.23,22.86
N$357  (via drill 1.07)
  other vias: 64.77,22.86
N$358  (via drill 1.07)
  other vias: 67.31,22.86
N$359  (via drill 1.07)
  other vias: 69.85,22.86
N$360  (via drill 1.07)
  other vias: 72.39,22.86
N$361  (via drill 1.07)
  other vias: 11.43,20.32
N$362  (via drill 1.07)
  other vias: 13.97,20.32
N$363  (via drill 1.07)
  other vias: 16.51,20.32
N$364  (via drill 1.07)
  other vias: 19.05,20.32
N$365  (via drill 1.07)
  other vias: 21.59,20.32
N$366  (via drill 1.07)
  other vias: 24.13,20.32
N$367  (via drill 1.07)
  other vias: 26.67,20.32
N$368  (via drill 1.07)
  other vias: 29.21,20.32
N$369  (via drill 1.07)
  other vias: 31.75,20.32
N$370  (via drill 1.07)
  other vias: 34.29,20.32
N$371  (via drill 1.07)
  other vias: 36.83,20.32
N$372  (via drill 1.07)
  other vias: 39.37,20.32
N$373  (via drill 1.07)
  other vias: 41.91,20.32
N$374  (via drill 1.07)
  other vias: 44.45,20.32
N$375  (via drill 1.07)
  other vias: 46.99,20.32
N$376  (via drill 1.07)
  other vias: 49.53,20.32
N$377  (via drill 1.07)
  other vias: 52.07,20.32
N$378  (via drill 1.07)
  other vias: 54.61,20.32
N$379  (via drill 1.07)
  other vias: 57.15,20.32
N$380  (via drill 1.07)
  other vias: 59.69,20.32
N$381  (via drill 1.07)
  other vias: 62.23,20.32
N$382  (via drill 1.07)
  other vias: 64.77,20.32
N$383  (via drill 1.07)
  other vias: 67.31,20.32
N$384  (via drill 1.07)
  other vias: 69.85,20.32
N$385  (via drill 1.07)
  other vias: 72.39,20.32
N$386  (via drill 1.07)
  other vias: 11.43,17.78
N$387  (via drill 1.07)
  other vias: 13.97,17.78
N$388  (via drill 1.07)
  other vias: 16.51,17.78
N$389  (via drill 1.07)
  other vias: 19.05,17.78
N$390  (via drill 1.07)
  other vias: 21.59,17.78
N$391  (via drill 1.07)
  other vias: 24.13,17.78
N$392  (via drill 1.07)
  other vias: 26.67,17.78
N$393  (via drill 1.07)
  other vias: 29.21,17.78
N$394  (via drill 1.07)
  other vias: 31.75,17.78
N$395  (via drill 1.07)
  other vias: 34.29,17.78
N$396  (via drill 1.07)
  other vias: 36.83,17.78
N$397  (via drill 1.07)
  other vias: 39.37,17.78
N$398  (via drill 1.07)
  other vias: 41.91,17.78
N$399  (via drill 1.07)
  other vias: 44.45,17.78
N$400  (via drill 1.07)
  other vias: 46.99,17.78
N$401  (via drill 1.07)
  other vias: 49.53,17.78
N$402  (via drill 1.07)
  other vias: 52.07,17.78
N$403  (via drill 1.07)
  other vias: 54.61,17.78
N$404  (via drill 1.07)
  other vias: 57.15,17.78
N$405  (via drill 1.07)
  other vias: 59.69,17.78
N$406  (via drill 1.07)
  other vias: 62.23,17.78
N$407  (via drill 1.07)
  other vias: 64.77,17.78
N$408  (via drill 1.07)
  other vias: 67.31,17.78
N$409  (via drill 1.07)
  other vias: 69.85,17.78
N$410  (via drill 1.07)
  other vias: 72.39,17.78
N$411  (via drill 1.07)
  other vias: 74.93,55.88
N$412  (via drill 1.07)
  other vias: 8.89,48.26
N$414  (via drill 1.07)
  other vias: 8.89,45.72
N$416  (via drill 1.07)
  other vias: 8.89,43.18
N$418  (via drill 1.07)
  other vias: 8.89,40.64
N$420  (via drill 1.07)
  other vias: 11.43,35.56
N$422  (via drill 1.07)
  other vias: 6.35,25.4
N$424  (via drill 1.07)
  other vias: 3.81,25.4
N$426  (via drill 1.07)
  other vias: 3.81,22.86
N$428  (via drill 1.07)
  other vias: 6.35,22.86
N$430  (via drill 1.07)
  other vias: 6.35,20.32
N$432  (via drill 1.07)
  other vias: 3.81,20.32
N$434  (via drill 1.07)
  other vias: 3.81,17.78
N$435  (via drill 1.07)
  other vias: 6.35,17.78
N$436  (via drill 1.07)
  other vias: 8.89,25.4
N$437  (via drill 1.07)
  other vias: 8.89,20.32
N$438  (via drill 1.07)
  other vias: 8.89,22.86
N$439  (via drill 1.07)
  other vias: 8.89,17.78
N$447  (via drill 1.07)
  other vias: 74.93,7.62
N$449  (via drill 1.07)
  other vias: 74.93,10.16
N$450  (via drill 1.07)
  other vias: 74.93,12.7
N$451  (via drill 1.07)
  other vias: 74.93,15.24
N$453  (via drill 1.07)
  other vias: 74.93,48.26
N$454  (via drill 1.07)
  other vias: 74.93,50.8
N$455  (via drill 1.07)
  other vias: 74.93,53.34

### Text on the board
tFinish: GND | GND | 51 | 41 | 35 | 33 | 30 | 27 | 24 | 22 | 17 | 15 | 12 | 10 | 8 | 6 | 2 | 144 | 142 | 140 | 138 | 134 | 132 | 127 | 124 | RAW | +V | 50 | 40 | 34 | 32 | 29 | 26 | 23 | 21 | 16 | 14 | 11 | 9 | 7 | 5 | 1 | 143 | 141 | 139 | 137 | 133 | 131 | 126 | 123 | AREF | GND | A9 | A8 | A7 | A6 | A5 | A4 | A1 | A0 | GND | GND | SUS | 58 | 67 | 75 | 79 | 81 | 83 | 85 | 88 | 93 | 95 | 98 | 100 | 102 | 105 | 112 | 115 | 117 | 119 | 121 | TMS | TDI | RST | RAW | +V | DONE | 57 | 66 | 74 | 78 | 80 | 82 | 84 | 87 | 92 | 94 | 97 | 99 | 101 | 104 | 111 | 114 | 116 | 118 | 120 | TDO | TCK | GND
bFinish: GND | GND | 51 | 41 | 35 | 33 | 30 | 27 | 24 | 22 | 17 | 15 | 12 | 10 | 8 | 6 | 2 | 144 | 142 | 140 | 138 | 134 | 132 | 127 | 124 | RAW | +V | 50 | 40 | 34 | 32 | 29 | 26 | 23 | 21 | 16 | 14 | 11 | 9 | 7 | 5 | 1 | 143 | 141 | 139 | 137 | 133 | 131 | 126 | 123 | AREF | GND | A9 | A8 | A7 | A6 | A5 | A4 | A1 | A0 | GND | GND | SUS | 58 | 67 | 75 | 79 | 81 | 83 | 85 | 88 | 93 | 95 | 98 | 100 | 102 | 105 | 112 | 115 | 117 | 119 | 121 | TMS | TDI | RST | RAW | +V | DONE | 57 | 66 | 74 | 78 | 80 | 82 | 84 | 87 | 92 | 94 | 97 | 99 | 101 | 104 | 111 | 114 | 116 | 118 | 120 | TDO | TCK | GND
